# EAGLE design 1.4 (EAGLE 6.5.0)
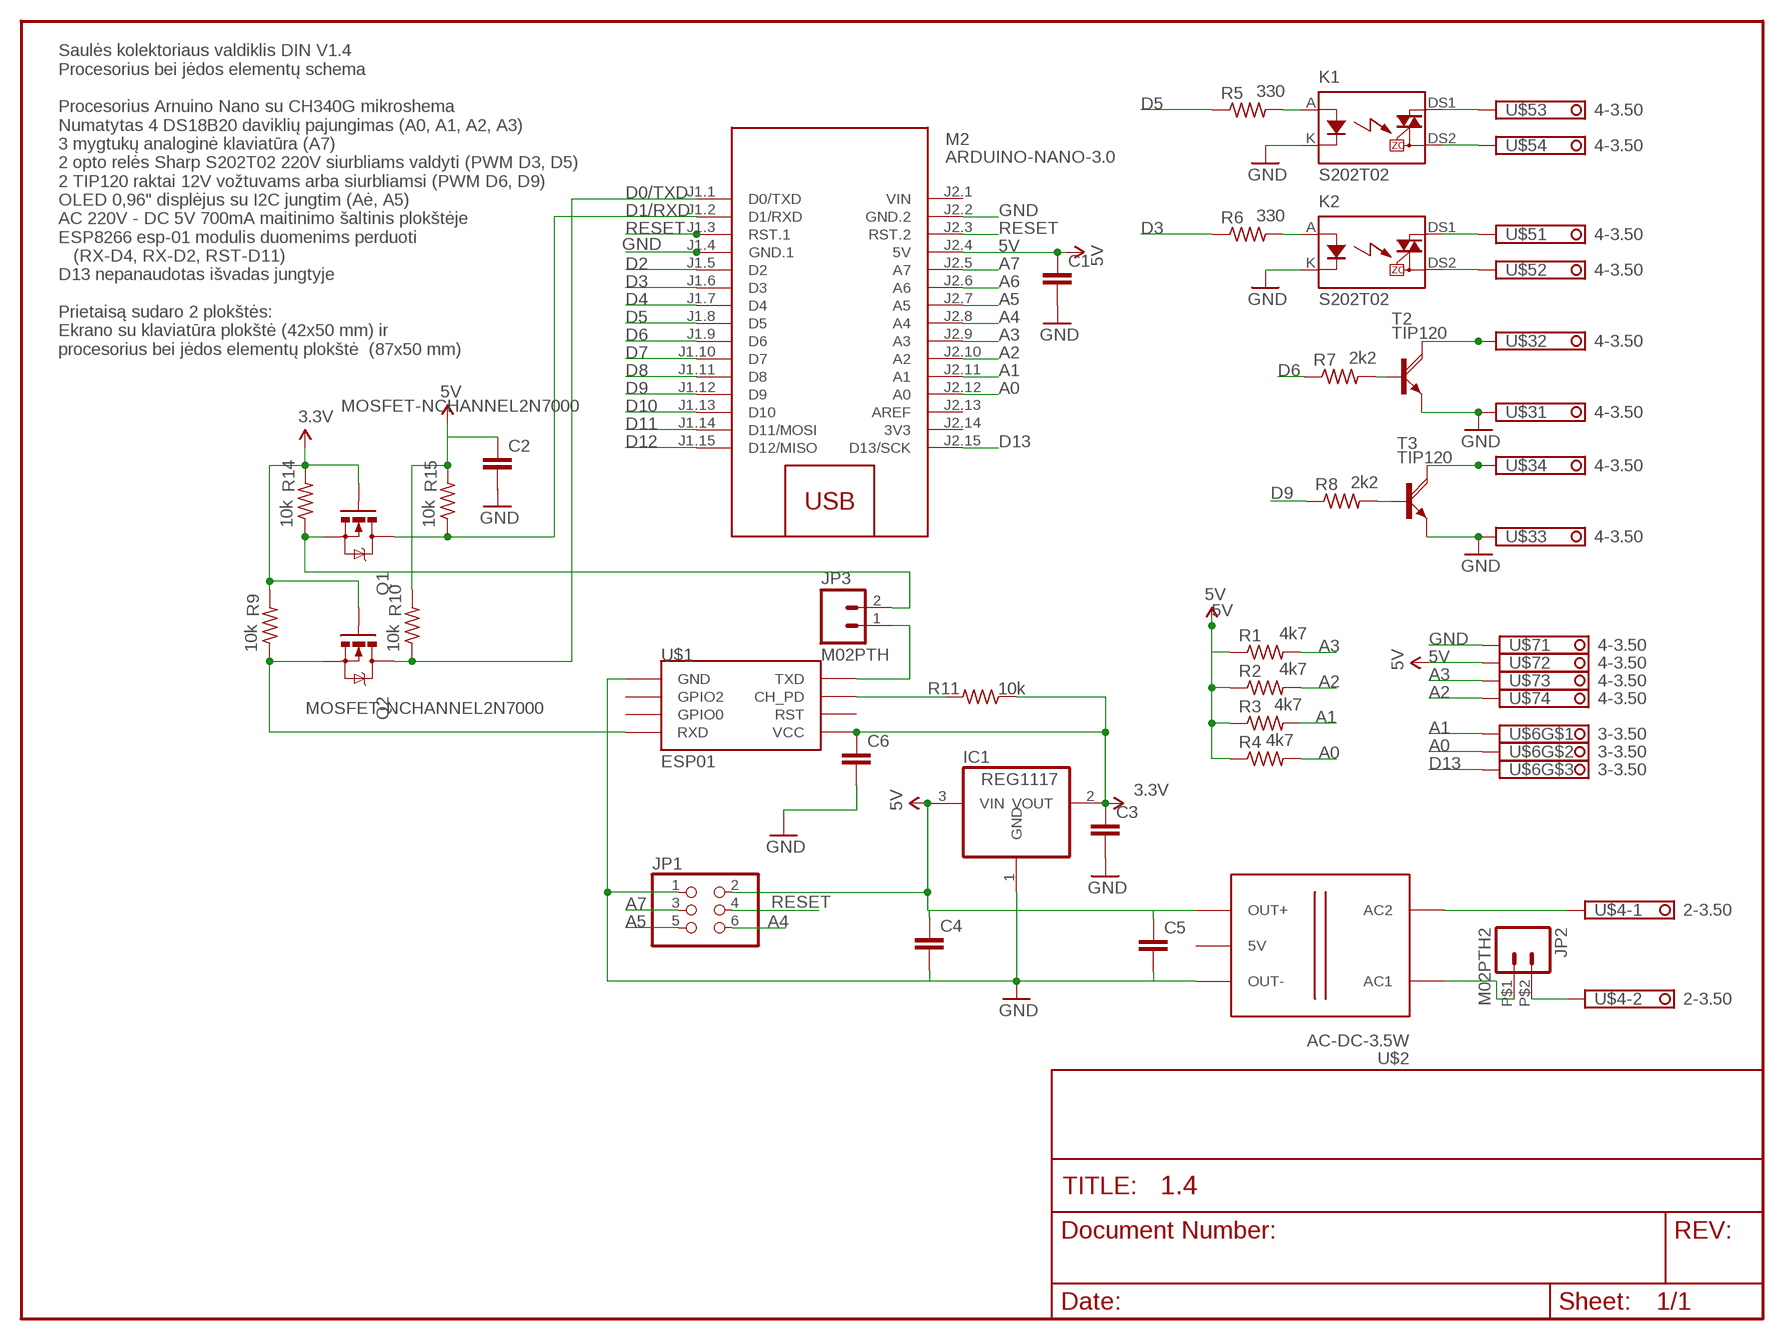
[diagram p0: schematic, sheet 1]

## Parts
C1  C-EU025-024X044  [C025-024X044]
C2  C-EU025-024X044  [C025-024X044]
C3  C-EU025-024X044  [C025-024X044]
C4  C-EU025-024X044  [C025-024X044]
C5  C-EU025-024X044  [C025-024X044]
C6  C-EU025-024X044  [C025-024X044]
IC1  REG1117  [SOT223]
JP1  PINHD-2X3  [2X03]
JP2  M02PTH2  [1X02_BIG]
JP3  M02PTH  [1X02]
K1  S202T02  [S202T02]
K2  S202T02  [S202T02]
M2  ARDUINO-NANO-3.0  [ARDUINO-NANO-3.0]
Q1  MOSFET-NCHANNEL2N7000  [TO-92]
Q2  MOSFET-NCHANNEL2N7000  [TO-92]
R1  4k7  R-US_0207/10  [0207/10]
R2  4k7  R-US_0207/10  [0207/10]
R3  4k7  R-US_0207/10  [0207/10]
R4  4k7  R-US_0207/10  [0207/10]
R5  330  R-US_0207/10  [0207/10]
R6  330  R-US_0207/10  [0207/10]
R7  2k2  R-US_0207/10  [0207/10]
R8  2k2  R-US_0207/10  [0207/10]
R9  10k  R-US_0207/10  [0207/10]
R10  10k  R-US_0207/10  [0207/10]
R11  10k  R-US_0207/10  [0207/10]
R14  10k  R-US_0207/10  [0207/10]
R15  10k  R-US_0207/10  [0207/10]
T2  TIP120  [TO220AH]
T3  TIP120  [TO220AH]
U$1  ESP01  [ESP01]
U$2  AC-DC-3.5W  [AC-DC-3.5W]
U$3  4-3.50  [4-3.50]
U$4  2-3.50  [2-3.50]
U$5  4-3.50  [4-3.50]
U$6  3-3.50  [3-3.50]
U$7  4-3.50  [4-3.50]

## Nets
3.3V: C3.1 C6.1 IC1.2(VOUT) Q1.2(G) Q2.2(G) R9.2 R11.1 R14.2 U$1.VCC
5V: C1.1 C2.1 C4.1 C5.1 IC1.3(VIN) JP1.2 M2.J2.4(5V) R1.1 R2.1 R3.1 R4.1 R10.2 R15.2 U$2.J2.3(OUT+) U$7.2
220V [220v]: U$2.J1.2(AC2) U$4.1
A0: M2.J2.12(A0) R4.2 U$6.2
A1: M2.J2.11(A1) R3.2 U$6.1
A2: M2.J2.10(A2) R2.2 U$7.4
A3: M2.J2.9(A3) R1.2 U$7.3
A4: JP1.6 M2.J2.8(A4)
A5: JP1.5 M2.J2.7(A5)
A6: M2.J2.6(A6)
A7: JP1.3 M2.J2.5(A7)
D0/TXD: M2.J1.1(D0/TXD) Q2.3(D) R10.1
D1/RXD: M2.J1.2(D1/RXD) Q1.3(D) R15.1
D2: M2.J1.5(D2)
D3: M2.J1.6(D3) R6.1
D4: M2.J1.7(D4)
D5: M2.J1.8(D5) R5.1
D6: M2.J1.9(D6) R7.1
D7: M2.J1.10(D7)
D8: M2.J1.11(D8)
D9: M2.J1.12(D9) R8.1
D10: M2.J1.13(D10)
D11: M2.J1.14(D11/MOSI)
D12: M2.J1.15(D12/MISO)
D13: M2.J2.15(D13/SCK) U$6.3
GND [220v]: C1.2 C3.2 C4.2 C5.2 C6.2 IC1.1(GND) JP1.1 K1.K K2.K M2.J1.4(GND.1) M2.J2.2(GND.2) T2.E T3.E U$1.GND U$2.J2.1(OUT-) U$3.1 U$3.3 U$7.1
N$1 [220v]: JP2.P$1 U$2.J1.1(AC1)
N$2 [220v]: JP2.P$2 U$4.2
N$3: R8.2 T3.B
N$4: R7.2 T2.B
N$5: K1.A R5.2
N$6: K2.A R6.2
N$7 [220v]: K1.DS1 U$5.3
N$8 [220v]: K1.DS2 U$5.4
N$9 [220v]: K2.DS2 U$5.2
N$10 [220v]: K2.DS1 U$5.1
N$12 [220v]: T2.C U$3.2
N$13: JP3.1 U$1.TX(TXD)
N$14 [220v]: T3.C U$3.4
N$16: R11.2 U$1.CH_PD
N$17: JP3.2 Q1.1(S) R14.1
N$18: Q2.1(S) R9.1 U$1.RX(RXD)
RESET: JP1.4 M2.J1.3(RST.1) M2.J2.3(RST.2)
Unconnected: C2.2 M2.J2.13(AREF) U$1.GPIO0 U$1.GPIO2 U$1.RST U$2.J2.2(5V)

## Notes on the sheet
- Saulės kolektoriaus valdiklis DIN V1.4
  Procesorius bei jėdos elementų schema
  
  Procesorius Arnuino Nano su CH340G mikroshema
  Numatytas 4 DS18B20 daviklių pajungimas (A0, A1, A2, A3)
  3 mygtukų analoginė klaviatūra (A7)
  2 opto relės Sharp S202T02 220V siurbliams valdyti (PWM D3, D5)
  2 TIP120 raktai 12V vožtuvams arba siurbliamsi (PWM D6, D9)
  OLED 0,96" displėjus su I2C jungtim (Aė, A5)
  AC 220V - DC 5V 700mA maitinimo šaltinis plokštėje
  ESP8266 esp-01 modulis duomenims perduoti
     (RX-D4, RX-D2, RST-D11)
  D13 nepanaudotas išvadas jungtyje
  
  Prietaisą sudaro 2 plokštės:
  Ekrano su klaviatūra plokštė (42x50 mm) ir 
  procesorius bei jėdos elementų plokštė  (87x50 mm)

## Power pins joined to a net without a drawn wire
3V3: M2.J2.14(3V3)
VIN: M2.J2.1(VIN)

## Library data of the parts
C1-C6 = rcl-1:C-EU: CAPACITOR, European symbol
IC1 = burr-brown:REG1117: 800mA and 1A Low Dropout (LDO) Positive Regulator 1.8V, 2.5V, 2.85V, 3.3V, 5V, and Adj; MPN: REG1117; OC_FARNELL: 1097566; OC_NEWARK: 14P6981
JP1 = pinhead-1:PINHD-2X3: PIN HEADER
JP2 = SparkFun-Connectors-1:M02: Standard 2-pin 0.1" header. Use with
JP3 = SparkFun-Connectors:M02: Standard 2-pin 0.1" header. Use with
K1 K2 = relay-1:S202T02
M2 = diy-modules-1:ARDUINO-NANO-3.0: Arduino Nano 3.0
Q1 Q2 = SparkFun-DiscreteSemi-1:MOSFET-NCHANNEL: Common NMOSFET Parts MFG P/NStore IDProd ID FDD8780TRANS-09984 SI7820DNTRANS-11055 FDS6630AIC-08089 2N7002PWTRANS-11151 FQP30N06L COM-10213TRANS-10060 BSS123LT1GTRANS-08345 BSS138TRANS-00830 BS170 2N7000
R1-R11 R14 R15 = resistor-1:R-US_: RESISTOR, American symbol
T2 T3 = rocketfarm:TIP120: NPN DARLINGTON TRANSISTOR
U$1 = esp8266modules-1:ESP01: ESP8266 Wifi module 01
U$2 = diy-modules-1:AC-DC-3.5W: AC/DC 3.5W Converter
U$3 U$5 U$7 = con-phoenix-350-1:4-3.50
U$4 = con-phoenix-350-1:2-3.50
U$6 = con-phoenix-350-1:3-3.50

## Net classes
0 default: width 0.5 mm
1 vcc: width 0.8 mm
2 +5v: width 0.8 mm
3 +3.3v: width 0.8 mm
4 gnd: width 1 mm
5 220v: width 1 mm

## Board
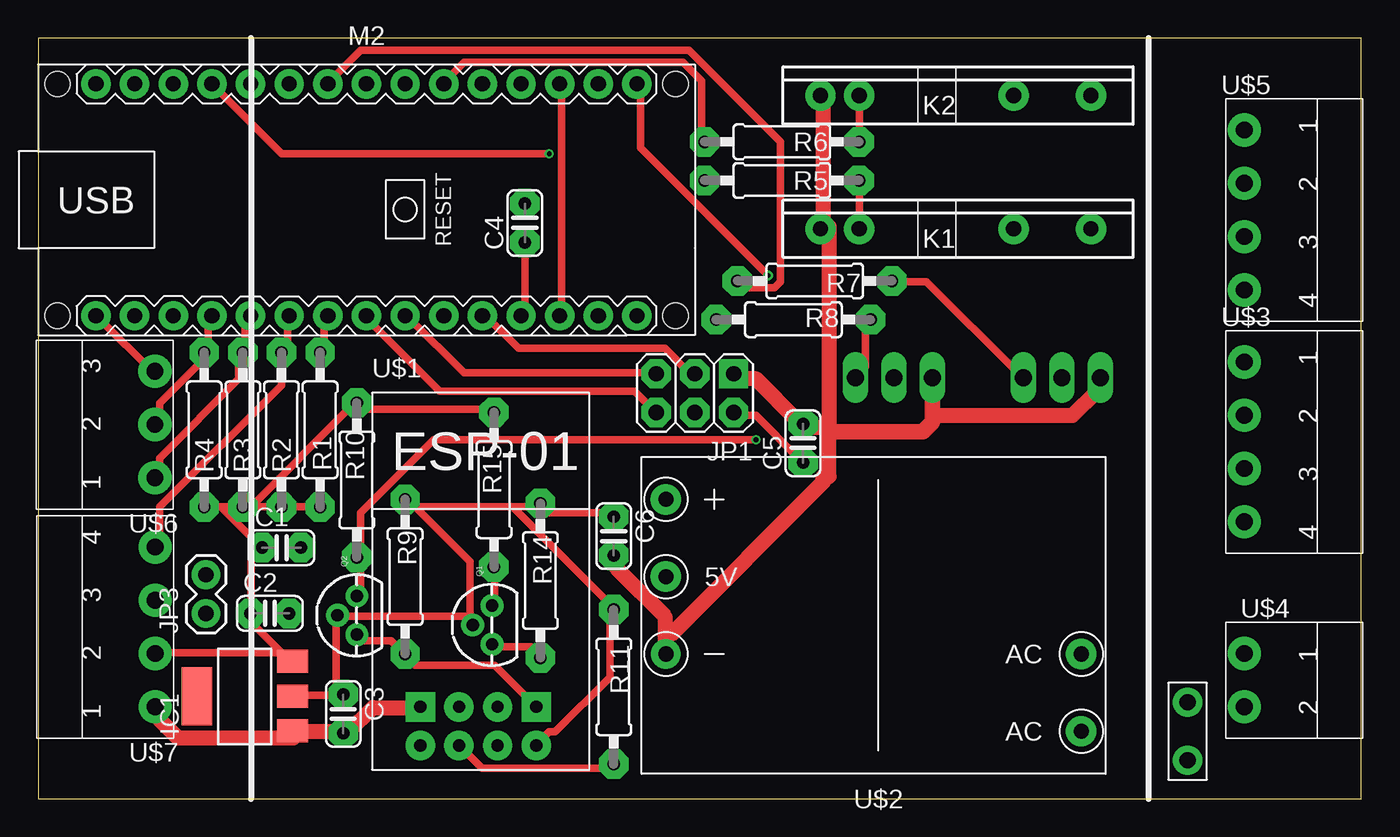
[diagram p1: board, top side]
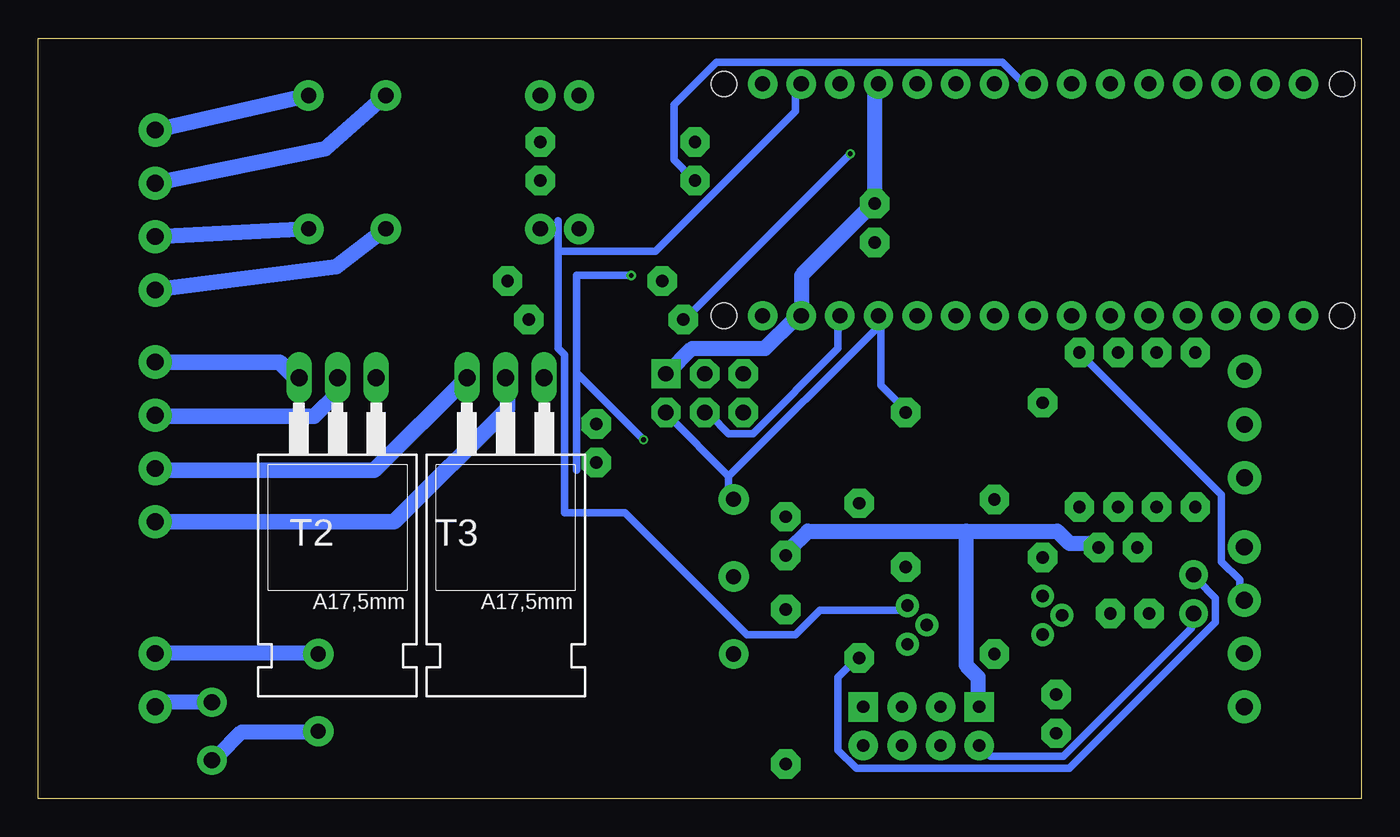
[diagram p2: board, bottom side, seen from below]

Size 87 x 50 mm. Coordinates in mm from the lower left corner, seen from the top.
Outline: 0,0 87,0 87,50 0,50 0,0
Copper layers (1*16): Top 0.035mm / dielectric 1.5mm / Bottom 0.035mm
Design rules "ITEADstudio_DRC": minimum track width 6mil, minimum drill 12mil, track to track 6mil, track to pad 6mil, pad to pad 6mil, via to via 6mil, smd to smd 0mil, copper to edge 10mil, drill to drill 10mil, minimum pad ring 10mil, minimum via ring 6mil, stop-mask expansion 2mil, vias tented up to drill 100mil, thermal gap 10mil

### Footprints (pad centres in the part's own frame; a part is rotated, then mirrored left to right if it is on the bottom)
C025-024X044 = drill 0.813 pad 1.93 octagon: 1 -1.27,0; 2 1.27,0
SOT223 = smd 1.499 x 2.007: 1 -2.261,-3.15; 2 0.025,-3.15; 3 2.311,-3.15 | smd 3.81 x 2.007: 4 0,3.15
2X03 = drill 1.016 pad 1.93 square: 1 -2.54,-1.27 | drill 1.016 pad 1.93 octagon: 2 -2.54,1.27; 3 0,-1.27; 4 0,1.27; 5 2.54,-1.27; 6 2.54,1.27
1X02_BIG = drill 1.067 pad 1.93: P$1 0,0; P$2 3.81,0
1X02 = drill 1.016 pad 1.88: 1 0,0; 2 2.54,0
S202T02 = drill 1 pad 2: A 10.16,0; DS1 -5.08,0; DS2 0,0; K 12.7,0
ARDUINO-NANO-3.0 = drill 1 pad 1.93: J1.1 17.78,7.62; J1.2 15.24,7.62; J1.3 12.7,7.62; J1.4 10.16,7.62; J1.5 7.62,7.62; J1.6 5.08,7.62; J1.7 2.54,7.62; J1.8 0,7.62; J1.9 -2.54,7.62; J1.10 -5.08,7.62; J1.11 -7.62,7.62; J1.12 -10.16,7.62; J1.13 -12.7,7.62; J1.14 -15.24,7.62; J1.15 -17.78,7.62; J2.1 17.78,-7.62; J2.2 15.24,-7.62; J2.3 12.7,-7.62; J2.4 10.16,-7.62; J2.5 7.62,-7.62; J2.6 5.08,-7.62; J2.7 2.54,-7.62; J2.8 0,-7.62; J2.9 -2.54,-7.62; J2.10 -5.08,-7.62; J2.11 -7.62,-7.62; J2.12 -10.16,-7.62; J2.13 -12.7,-7.62; J2.14 -15.24,-7.62; J2.15 -17.78,-7.62 | hole 1.651: -20.32,7.62; -20.32,-7.62; 20.32,-7.62; 20.32,7.62
TO-92 = drill 0.813 pad 1.5: 1 -1.27,0; 2 0,1.27; 3 1.27,0
0207/10 = drill 0.813 pad 1.93 octagon: 1 -5.08,0; 2 5.08,0
TO220AH = drill 1.118 long: B -2.54,-6.35; C 0,-6.35; E 2.54,-6.35
ESP01 = drill 0.8 pad 1.93: CH_PD -1.285,-8.178; GPIO0 1.255,-5.638; GPIO2 -1.285,-5.638; RST 1.255,-8.178; TX -3.825,-8.178; VCC 3.795,-8.178 | drill 0.8 pad 1.93 square: GND -3.825,-5.638; RX 3.795,-5.638
AC-DC-3.5W = drill 1 pad 2: J1.1 -13.335,7.62; J1.2 -13.335,2.54; J2.2 13.97,-2.54; J2.3 13.97,-7.62 | drill 1 pad 1.93: J2.1 13.97,2.54
4-3.50 = drill 1.1 pad 2.184: 1 2.05,1.2; 2 5.55,1.2; 3 9.05,1.2; 4 12.55,1.2
2-3.50 = drill 1.1 pad 2.184: 1 2.05,1.2; 2 5.55,1.2
3-3.50 = drill 1.1 pad 2.184: 1 2.05,1.2; 2 5.55,1.2; 3 9.05,1.2

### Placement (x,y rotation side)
C1  16,16.51 0 top
C2  15.24,12.19 0 top
C3  20.07,5.59 270 top
C4  32,37.85 90 top
C5  50.29,23.37 90 top
C6  37.85,17.27 270 top
IC1  13.59,6.73 90 top
JP1  43.18,26.67 180 top
JP2  75.56,2.54 90 top
JP3  11.05,12.19 90 top
K1  64.14,37.47 180 top
K2  64.14,46.23 180 top
M2  21.59,39.37 0 top
Q1  29.84,11.43 90 top
Q2  20.95,12.06 90 top
R1  18.54,24.26 90 top
R2  16,24.26 90 top
R3  13.46,24.26 90 top
R4  10.92,24.26 90 top
R5  48.9,40.64 0 top
R6  48.9,43.18 0 top
R7  51.05,34.04 0 top
R8  49.66,31.5 0 top
R9  24.13,14.61 90 top
R10  20.95,20.95 90 top
R11  37.85,7.37 270 top
R14  33.02,14.35 90 top
R15  29.97,20.32 90 top
T2  67.31,21.34 180 bottom
T3  56.26,21.34 180 bottom
U$1  28.96,11.68 0 top
U$2  55.24,12.06 180 top
U$3  78.09,30.76 270 top
U$4  78.09,11.6 270 top
U$5  78.09,46 270 top
U$6  8.89,19.05 90 top
U$7  8.9,4 90 top

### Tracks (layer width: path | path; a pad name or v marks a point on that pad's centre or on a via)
3.3V
  Top 0.5: U$1.VCC 32.8,3.6 33.6,4.4 34,4.4 37.6,8 37.6,12.4 R11.1 37.6,12.8 31.2,19.2 | 19.6,6.8 20,6.8 C3.1 19.6,6.8 | 19.6,6.8 16.8,6.8 IC1.2 | 19.6,6.8 19.6,12 Q2.2 20,12 28.4,12 | 28.4,12 28.4,15.6 24.8,19.2 | 28.4,12 28.4,11.6 Q1.2 28.4,12 | 24.8,19.2 24.4,19.6 R9.2 24.8,19.2 | 24.8,19.2 31.2,19.2 | 31.2,19.2 32.8,19.2 R14.2 33.2,19.2 33.6,18.8 37.6,18.8 C6.1
5V
  Top 0.5: C5.1 50,22.4 47.2,25.2 46,25.2 JP1.2 | 16,9.6 13.6,12 C2.1 14,12.4 14,17.2 | 16,9.6 16.4,9.2 IC1.3 16,9.6 | 16,9.6 8,9.6 U$7.2 | M2.J2.4 32,32 32,36.4 C4.1 | R1.1 18.4,19.2 16.4,19.2 R2.1 16,19.2 14,19.2 | 12,19.2 13.2,19.2 R3.1 | 12,19.2 11.2,19.2 R4.1 | 12,19.2 14,17.2 | 14,17.2 14.4,16.8 C1.1 | 14,19.2 13.6,18.8 R3.1 | 14,19.2 20.4,25.6 | 20.4,25.6 20.8,26 R10.2 20.4,25.6 | 20.4,25.6 29.6,25.6 R15.2 | 14,19.2 R3.1
  Bottom 0.5: 41.6,21.2 41.6,20 U$2.J2.3 | 41.6,21.2 45.6,25.2 JP1.2 | 31.6,31.2 31.6,27.2 30,25.6 R15.2 | 31.6,31.2 31.6,31.6 M2.J2.4 31.6,31.2 | 31.6,31.2 41.6,21.2
220V
  Bottom 1: U$2.J1.2 68.8,9.6 79.2,9.6 U$4.1
A0
  Top 0.5: M2.J2.12 11.2,31.6 11.2,29.6 R4.2 11.2,29.2 8,26 8,24.8 U$6.2
A1
  Top 0.5: M2.J2.11 13.6,31.6 13.6,29.6 R3.2 13.2,29.2 13.2,27.6 8,22.4 8,21.2 U$6.1
A2
  Top 0.5: M2.J2.10 16.4,31.6 16.4,29.6 R2.2 16,29.2 16,27.2 8,19.2 8,16.8 U$7.4
A3
  Top 0.5: R1.2 18.8,29.6 18.8,31.6 M2.J2.9
  Bottom 0.5: U$7.3 8,13.2 8,14.4 9.2,15.6 9.2,20 18.4,29.2 R1.2
A4
  Top 0.5: M2.J2.8 21.6,31.6 26.4,26.8 39.2,26.8 40.4,25.6 JP1.6
A5
  Top 0.5: M2.J2.7 24.4,31.6 28,28 40.4,28 JP1.5
A7
  Top 0.5: M2.J2.5 29.6,31.6 31.6,29.6 41.2,29.6 42.8,28 JP1.3
D0/TXD  (via drill 0.3)
  Top 0.5: Q2.3 21.2,13.6 21.2,15.6 R10.1 21.2,16 21.2,18.8 26,23.6 v47.2,23.6 | v48,34.4 39.6,42.8 39.6,46.8 M2.J1.1
  Bottom 0.5: 51.6,28 51.6,34.4 v48,34.4 | 51.6,28 51.6,21.6 | 51.6,28 v47.2,23.6
D1/RXD
  Top 0.5: Q1.3 30,12.8 30,15.2 R15.1
  Bottom 0.5: 52.8,36 52.8,29.6 52.4,29.2 52.4,18.8 48.4,18.8 40.4,10.8 37.2,10.8 35.6,12.4 30,12.4 Q1.3 | 52.8,36 52.8,38 | 52.8,36 46.4,36 37.2,45.2 37.2,46.8 M2.J1.2
D3
  Top 0.5: M2.J1.6 26.8,47.2 28,48.4 42.4,48.4 43.6,47.2 43.6,43.2 R6.1
D5
  Bottom 0.5: M2.J1.8 21.6,47.2 22.4,47.2 23.6,48.4 42.4,48.4 45.2,45.6 45.2,42 44,40.8 R5.1
D6
  Top 0.5: M2.J1.9 19.2,47.2 21.2,49.2 42.8,49.2 48.8,43.2 48.8,34 48.4,33.6 46.4,33.6 46,34 R7.1
D9  (via drill 0.3)
  Top 0.5: v33.6,42.4 16,42.4 11.6,46.8 M2.J1.12
  Bottom 0.5: v33.6,42.4 44.4,31.6 R8.1
D13
  Top 0.5: M2.J2.15 4,31.6 7.6,28 U$6.3
GND
  Top 1: K2.K 51.6,46 51.6,37.6 K1.K 52,37.6 52,24.13 | 58.8,25.2 68,25.2 69.6,26.8 69.6,27.6 T2.E | 52,24.13 52,21.2 51.6,21.2 51.6,20.8 41.6,10.8 41.2,10.8 | 16.8,4.4 IC1.1 | IC1.1 17.2,4.4 20,4.4 C3.2 20.4,4.4 22,6 24.8,6 U$1.GND | U$7.1 8,6 8,5.2 9.2,4 16.8,4 IC1.1 | JP1.1 46,27.6 47.2,27.6 50,24.8 C5.2 50.4,24.4 51.6,24.4 52,24.13 | 41.2,10.8 41.2,12 38,15.2 38,16 C6.2 | 41.2,10.8 41.2,9.6 U$2.J2.1
  Top 1.016: T3.E 58.8,25.2 58.8,24.77 58.17,24.13 52,24.13
  Bottom 1: M2.J1.4 32,46.8 32,39.2 C4.2 32.4,38.8 36.8,34.4 36.8,32 M2.J2.2 37.2,31.6 39.2,29.6 44,29.6 45.6,28 JP1.1 | 26,17.6 36.4,17.6 37.6,16.4 C6.2 | 26,17.6 20,17.6 19.2,16.8 17.6,16.8 C1.2 | 26,17.6 26,8.8 25.2,8 25.2,6.4 U$1.GND
  Bottom 1.016: U$3.3 79.17,21.59 64.9,21.59 T3.E | U$3.1 79.29,28.7 71.12,28.7 70.1,27.69 T2.E
N$1
  Bottom 1: U$2.J1.1 68.8,4.4 73.6,4.4 75.2,2.8 JP2.P$1
N$2
  Bottom 1: JP2.P$2 75.6,6.4 79.2,6.4 U$4.2
N$3
  Top 0.5: R8.2 54.4,31.2 54.4,28.4 54,28 T3.B
N$4
  Top 0.5: R7.2 56.4,34 58.4,34 64.4,28 T2.B
N$5
  Top 0.5: R5.2 54,40.4 54,37.6 K1.A
N$6
  Top 0.5: R6.2 54,43.2 54,46 K2.A
N$7
  Bottom 1.016: U$5.3 K1.DS1
N$8
  Bottom 1.016: U$5.4 67.39,34.97 K1.DS2
N$9
  Bottom 1.016: U$5.2 68.14,42.74 K2.DS2
N$10
  Bottom 1.016: U$5.1 K2.DS1
N$12
  Bottom 1.016: U$3.2 79.23,25.15 68.83,25.15 67.31,26.67 T2.C
N$13
  Bottom 0.5: JP3.1 11.2,12 11.2,11.2 19.6,2.8 24.4,2.8 24.8,3.2 U$1.TX
N$14
  Bottom 1.016: U$3.4 63.58,18.21 56.13,25.65 56.13,27.56 T3.C
N$16
  Top 0.5: U$1.CH_PD 28,3.2 29.2,2 37.6,2 R11.2
N$17
  Top 0.5: Q1.1 30,10 32.4,10 32.8,9.6 R14.1
  Bottom 0.5: JP3.2 10.8,14.4 9.6,13.2 9.6,11.6 19.2,2 33.2,2 34.4,3.2 34.4,8 33.2,9.2 R14.1
N$18
  Top 0.5: Q2.1 21.2,10.4 23.2,10.4 24,9.6 R9.1 24.4,9.2 24.8,8.8 30,8.8 32.4,6.4 U$1.RX
RESET
  Top 0.5: M2.J2.3 34.4,32 34.4,46.8 M2.J1.3
  Bottom 0.5: JP1.4 42.8,25.2 41.6,24 40,24 34.4,29.6 34.4,31.6 M2.J2.3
